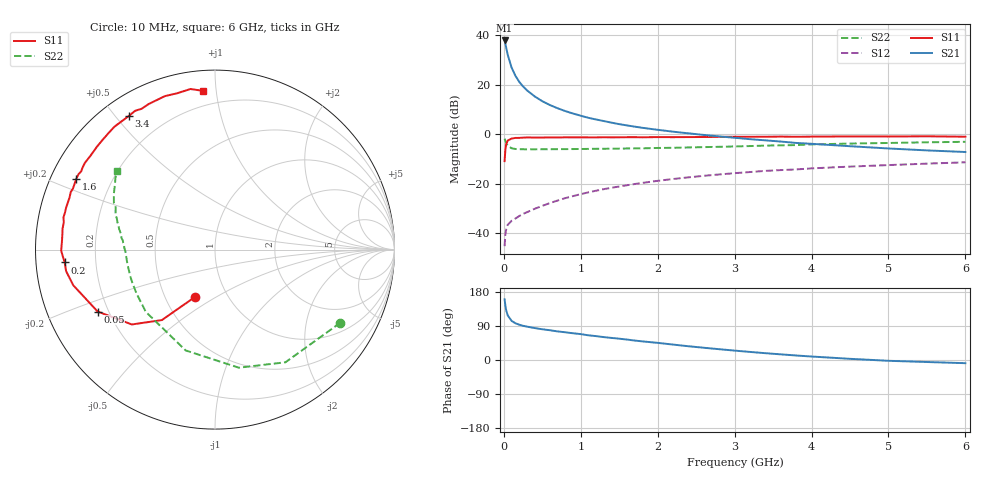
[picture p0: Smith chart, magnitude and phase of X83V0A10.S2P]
! SIEMENS Small Signal Semiconductors
! BFP136W
! Si NPN RF Bipolar Junction Transistor in SOT343
! VCE = 3 V  IC = 100 mA
! Common Emitter S-Parameters:  September  1994
# GHz  S  MA  R  50
!  f  S11  S21  S12  S22
! GHz  MAG  ANG  MAG  ANG  MAG  ANG  MAG  ANG
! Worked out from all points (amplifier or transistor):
!   40 points, 10 MHz to 6 GHz, reference 50 ohm
!   highest |S21| = 37.9 dB at 10 MHz (marker M1)
!   |S21| within 3 dB of that: start of sweep to 31.26 MHz
!   unconditionally stable (mu >= 1): 506.1 MHz to 2.887 GHz
!   at 200 MHz: K = 0.70, MSG = 27.2 dB, |S12| = -33.2 dB
!   at 1.5 GHz: K = 1.11, MAG = 10.6 dB, |S12| = -21.2 dB
!   at 6 GHz: K = 0.98, MSG = 2.1 dB, |S12| = -11.4 dB
!   S11 on the Smith chart (normalised r, x): 10 MHz: 0.71, -0.40; 50 MHz: 0.16, -0.24; 200 MHz: 0.09, -0.04; 1.6 GHz: 0.08, +0.24; 3.4 GHz: 0.08, +0.54; 6 GHz: 0.11, +0.92
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0.01  0.2841 -112.6  78.82 160.2  0.0054 69.4  0.8084 -30.3
0.02  0.4916 -127.0  67.61 143.6  0.0096 56.1  0.7404 -58.0
0.03  0.6234 -138.0  57.01 131.9  0.0117 49.4  0.6712 -78.6
0.05  0.7395 -152.2  40.57 117.8  0.0146 40.4  0.5851 -106.2
0.1  0.8145 -165.9  22.41 103.4  0.0176 36.7  0.5186 -138.0
0.15  0.8383 -171.8  15.24 97.0  0.0196 39.9  0.5008 -151.1
0.2  0.8406 -175.1  11.46 93.2  0.022 42.6  0.4961 -158.3
0.25  0.85 -177.8  9.241 90.2  0.0243 45.2  0.495 -162.8
0.3  0.857 -179.6  7.732 88.1  0.0263 47.5  0.4934 -165.9
0.4  0.8539 176.9  5.82 84.3  0.0308 51.5  0.4942 -170.0
0.5  0.8547 174.3  4.64 81.1  0.0353 54.6  0.495 -172.8
0.6  0.8573 172.2  3.875 78.5  0.0404 56.7  0.4954 -174.6
0.7  0.856 169.7  3.338 75.4  0.0454 58.8  0.4969 -176.0
0.9  0.8608 166.2  2.612 70.5  0.0557 60.1  0.499 -178.6
1.1  0.8606 161.7  2.139 65.1  0.0664 60.6  0.5029 179.8
1.6  0.8674 153.1  1.503 54.0  0.0924 59.5  0.5129 175.8
2.2  0.8687 142.8  1.122 40.7  0.1236 55.2  0.5292 171.2
3.2  0.8841 126.1  0.791 21.3  0.171 45.8  0.5738 162.4
3.4  0.8857 122.9  0.749 18.0  0.1805 43.7  0.5867 160.7
4.5  0.8995 108.1  0.57 3.1  0.2204 33.5  0.6448 150.9
5.5  0.9052 98.7  0.469 -5.3  0.253 25.6  0.684 144.2
6  0.8871 94.4  0.435 -8.4  0.2694 21.3  0.6995 141.3
